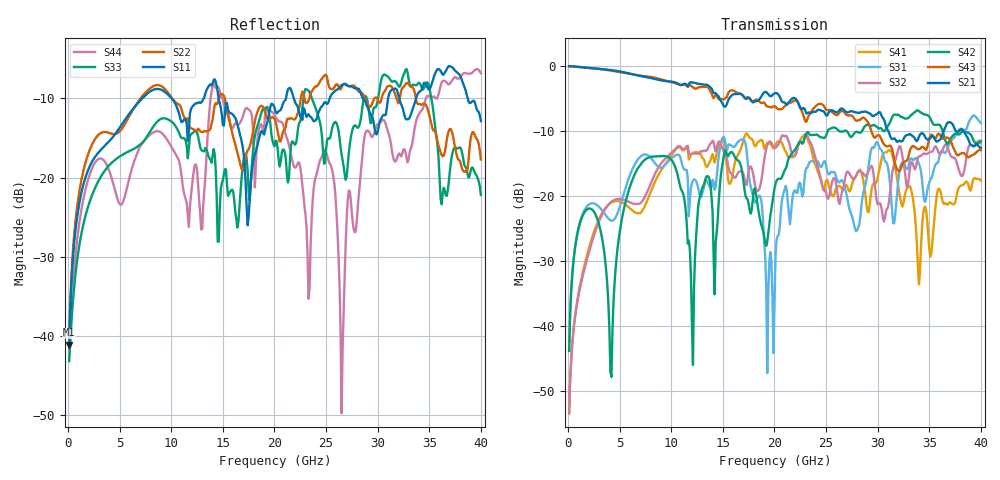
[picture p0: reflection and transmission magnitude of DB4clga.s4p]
! ADC12DJ3200QML-SP
! 196-pin ZMX package
! CLGA Ceramic Package without columns (ceramic land grid array)
! Texas Instruments 4/21/2021
! Single-ended  S-parameters
! PORT#  PORT_NAME  NET_NAME
! PORT1:  DAxN.DIEBUMP DAxN
! PORT2:  DAxN.BGA  DAxN
! PORT3:  DAxP.DIEBUMP DAxP
! PORT4:  DAxP.BGA  DAxP
! Touchstone Ver. 1.0
! Number of ports is 4
# Hz	S	MA	R	50.000000
! SCATTERING PARAMETERS  :
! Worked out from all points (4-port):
!   400 points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, 100 MHz to 40 GHz, reference 50 ohm
!   strongest paths, dB at 100 MHz, 10.1 GHz, 20.1 GHz, 30.1 GHz, 40 GHz:
!     S21: -0.1, -2.5, -4.2, -7.2, -12.6
!     S43: -0.1, -2.5, -6.3, -10.7, -13.0
!     S42: -43.8, -14.7, -18.1, -9.6, -11.5
!     S32: -53.4, -13.3, -12.6, -21.2, -11.9
!     S31: -43.8, -14.1, -29.3, -12.3, -8.8
!     S41: -53.4, -13.6, -12.2, -16.4, -17.6
!   lowest |S11| = -41.2 dB at 100 MHz (marker M1), VSWR 1.02, Z = 50.6 - j0.651 ohm
!   |S11| at or under -10 dB: start of sweep to 7.186 GHz; 14.58 GHz to 21.12 GHz (6.533 GHz wide, 36.6 % of centre); 21.88 GHz to 25.35 GHz (3.478 GHz wide, 14.7 % of centre)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
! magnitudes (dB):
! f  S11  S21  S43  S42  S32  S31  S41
! 100 MHz  -41.2  -0.1  -0.1  -43.8  -53.4  -43.8  -53.4
! 10.6 GHz  -11.3  -2.7  -2.8  -16.7  -12.5  -13.7  -12.4
! 12.1 GHz  -10.9  -2.6  -3.3  -46.0  -13.5  -17.6  -13.4
! 19.3 GHz  -13.0  -4.2  -6.3  -27.1  -12.2  -47.2  -11.9
! 26.5 GHz  -8.3  -6.6  -6.9  -10.1  -19.7  -17.6  -18.9
! 28.8 GHz  -10.3  -7.0  -8.2  -9.2  -17.0  -18.4  -19.6
! 40 GHz  -12.9  -12.6  -13.0  -11.5  -11.9  -8.8  -17.6
